[IBIS Ver]   4.0
[Comment Char] |_char
[File name]   pse84_ewlb235.ibs
[File Rev] 1.2
[Date] 10/27/2023
[Source] Infineon Technologies IBIS team
[Notes]
|Rev. 1.0 - Initial model 12/8/2021
|Rev. 1.1 - Update with RLC 8/19/2023
|Rev. 1.2 - Included pins for MIPI-DPHY DSI and USB 10/23/2023
|The temperature range is -40 to 125C.
|This model was syntax checked with Hyperlynx 4.2 visual IBIS
|editor and ibischk7_64 IBIS checker.
|There were 0 syntax errors.
[Disclaimer]   The model given below represents a 235-pin package.
[Copyright]   (C) COPYRIGHT 2023, Infineon Technologies AG.
[Component] PSOCE84
[Manufacturer] Infineon Technologies AG
| Package model eWLB235 was extracted from simulation tool.
[Package]
|   typ   min   max
R_pkg   0.27855   0.02289   0.76353
L_pkg   0.886n   0.101n   2.38n
C_pkg   0.191p   0.0717p   0.401p
[Pin]   Signal_name   model_name   R_pin   L_pin   C_pin
A10   P16_1_PAD   3p3_gpio_wbso_v 0.40002 1.87E-09   1.65E-13
A8   P17_5_PAD   3p3_gpio_wbso_v 0.60238 2.38E-09   2.00E-13
B8   P17_3_PAD   3p3_gpio_wbso_v 0.42798 1.66E-09   1.54E-13
C10   P16_3_PAD   3p3_gpio_wbso_v 0.31957 1.40E-09   1.50E-13
D7   P17_7_PAD   3p3_gpio_wbso_v 0.43638 8.69E-10   2.95E-13
E9   P16_7_PAD   3p3_gpio_wbso_v 0.45335 8.89E-10   2.99E-13
G7   P17_1_PAD   3p3_gpio_wbso_v 0.66331 1.27E-09   3.60E-13
G8   P16_5_PAD   3p3_gpio_wbso_v 0.65241 1.26E-09   3.71E-13
B10   P16_2_PAD   3p3_gpio_wbso_v 0.34579 1.53E-09   1.69E-13
B11   P16_0_PAD   3p3_gpio_wbso_v 0.28083 1.31E-09   1.32E-13
C7   P17_6_PAD   3p3_gpio_wbso_v 0.43877 1.72E-09   1.62E-13
C8   P17_4_PAD   3p3_gpio_wbso_v 0.36424 1.41E-09   1.67E-13
E7   P17_2_PAD   3p3_gpio_wbso_v 0.46653 9.28E-10   3.04E-13
E8   P17_0_PAD   3p3_gpio_wbso_v 0.39239 7.88E-10   2.83E-13
F8   P16_6_PAD   3p3_gpio_wbso_v 0.55142 1.07E-09   3.42E-13
F9   P16_4_PAD   3p3_gpio_wbso_v 0.47491 9.43E-10   3.06E-13
R10   XRES_PAD   1p8_xres_3swbso 0.029075   2.89E-10   7.84E-14
J10   P11_5_PAD   1p8_ovt_wbso_h  0.59768 1.17E-09   3.42E-13
K11   P11_3_PAD   1p8_ovt_wbso_h  0.43593 8.51E-10   3.12E-13
K12   P11_4_PAD   1p8_ovt_wbso_h  0.34228 6.90E-10   2.69E-13
K13   P11_6_PAD   1p8_ovt_wbso_h  0.24957 5.13E-10   2.42E-13
K15   P11_7_PAD   1p8_ovt_wbso_h  0.028195   1.17E-10   1.82E-13
K16   P11_1_PAD   1p8_ovt_wbso_h  0.07529 4.02E-10   7.83E-14
L11   P11_2_PAD   1p8_ovt_wbso_h  0.43058 8.35E-10   3.10E-13
L16   P11_0_PAD   1p8_ovt_wbso_h  0.02734 1.88E-10   7.18E-14
H7   P3_0_PAD   1p8_ioi3c_3swbso_h   0.39265 8.57E-10   3.36E-13
H8   P3_1_PAD   1p8_ioi3c_3swbso_h   0.46598 1.05E-09   3.57E-13
A14   P20_4_PAD   1p8_ioi2c_wbso_h   0.23793 1.20E-09   1.02E-13
B12   P20_6_PAD   1p8_ioi2c_wbso_h   0.18255 9.43E-10   9.44E-14
B14   P20_2_PAD   1p8_ioi2c_wbso_h   0.14411 7.56E-10   8.93E-14
B15   P20_0_PAD   1p8_ioi2c_wbso_h   0.1456  7.01E-10   9.21E-14
E12   P9_2_PAD   1p8_ioi2c_wbso_h   0.25292 5.97E-10   2.66E-13
F10   P9_0_PAD   1p8_ioi2c_wbso_h   0.66966 1.28E-09   3.71E-13
K9   P8_7_PAD   1p8_ioi2c_wbso_h   0.47076 9.33E-10   3.06E-13
M8   P8_6_PAD   1p8_ioi2c_wbso_h   0.21737 4.56E-10   2.33E-13
R8   P8_2_PAD   1p8_ioi2c_wbso_h   0.039885 3.42E-10   7.77E-14
T6   P8_4_PAD   1p8_ioi2c_wbso_h   0.36053 1.26E-09   1.31E-13
T7   P8_5_PAD   1p8_ioi2c_wbso_h   0.17838 7.65E-10   9.60E-14
U6   P8_3_PAD   1p8_ioi2c_wbso_h   0.40499 1.49E-09   1.31E-13
A2   P6_4_PAD   1p8_ioi2c_wbso_h   0.31511 1.29E-09   1.19E-13
B2   P6_6_PAD   1p8_ioi2c_wbso_h   0.2468  1.02E-09   1.15E-13
K8   P21_4_PAD   1p8_ioi2c_wbso_h   0.6339  1.22E-09   3.78E-13
L12   P10_1_PAD   1p8_ioi2c_wbso_h   0.2568  6.95E-10   3.15E-13
M15   P10_2_PAD   1p8_ioi2c_wbso_h   0.022894 1.01E-10   1.82E-13
M4   P21_6_PAD   1p8_ioi2c_wbso_h   0.089229 2.15E-10   1.97E-13
P16   P10_3_PAD   1p8_ioi2c_wbso_h   0.31745 1.26E-09   1.37E-13
P4   P12_0_PAD   1p8_ioi2c_wbso_h   0.083721 2.60E-10   2.03E-13
R2   P21_2_PAD   1p8_ioi2c_wbso_h   0.29537 1.18E-09   1.23E-13
T16   P10_0_PAD   1p8_ioi2c_wbso_h   0.26089 1.05E-09   1.83E-13
T2   P21_0_PAD   1p8_ioi2c_wbso_h   0.37991 1.33E-09   1.56E-13
T3   P12_2_PAD   1p8_ioi2c_wbso_h   0.22827 9.38E-10   1.27E-13
U2   P12_4_PAD   1p8_ioi2c_wbso_h   0.34327 1.27E-09   1.28E-13
A12   P20_5_PAD   1p8_ioi2c_wbso_h   0.27304 1.32E-09   1.10E-13
A16   P20_1_PAD   1p8_ioi2c_wbso_h   0.31259 1.50E-09   1.18E-13
C12   P20_7_PAD   1p8_ioi2c_wbso_h   0.15854 7.92E-10   9.47E-14
C14   P20_3_PAD   1p8_ioi2c_wbso_h   0.064528 3.41E-10   8.12E-14
F11   P9_1_PAD   1p8_ioi2c_wbso_h   0.48015 9.35E-10   3.18E-13
G9   P9_3_PAD   1p8_ioi2c_wbso_h   0.71533 1.38E-09   3.75E-13
B1   P6_7_PAD   1p8_ioi2c_wbso_h   0.35877 1.34E-09   1.24E-13
B3   P6_5_PAD   1p8_ioi2c_wbso_h   0.22409 8.52E-10   1.02E-13
L7   P21_7_PAD   1p8_ioi2c_wbso_h   0.39102 7.76E-10   2.88E-13
L8   P21_3_PAD   1p8_ioi2c_wbso_h   0.5432  1.04E-09   3.65E-13
M5   P21_5_PAD   1p8_ioi2c_wbso_h   0.19144 3.96E-10   2.31E-13
R3   P12_5_PAD   1p8_ioi2c_wbso_h   0.066979 4.06E-10   8.45E-14
R4   P12_1_PAD   1p8_ioi2c_wbso_h   0.15282 5.87E-10   1.11E-13
T1   P21_1_PAD   1p8_ioi2c_wbso_h   0.4827  1.76E-09   1.69E-13
U3   P12_3_PAD   1p8_ioi2c_wbso_h   0.30929 1.38E-09   1.36E-13
A3   P6_3_PAD   1p8_ioi2c_wbso_h   0.17141 1.04E-09   1.16E-13
A4   P6_2_PAD   1p8_ioi2c_wbso_h   0.17085 1.05E-09   1.16E-13
B4   P6_1_PAD   1p8_ioi2c_wbso_h   0.1086  6.90E-10   8.90E-14
C6   P6_0_PAD   1p8_ioi2c_wbso_h   0.16176 7.51E-10   1.29E-13
K10   P8_0_PAD   1p8_ioi2c_wbso_h   0.60411 1.17E-09   3.43E-13
T8   P8_1_PAD   1p8_ioi2c_wbso_h   0.093729 6.77E-10   9.47E-14
B17   P15_6_PAD   1p8_ioi2c_wbso_h   0.20398 1.14E-09   1.22E-13
C16   P15_7_PAD   1p8_ioi2c_wbso_h   0.067252 4.46E-10   9.19E-14
D17   P15_5_PAD   1p8_ioi2c_wbso_h   0.070339 5.96E-10   8.57E-14
D5   P7_0_PAD   1p8_ioi2c_wbso_h   0.11478 3.74E-10   2.53E-13
D6   P7_1_PAD   1p8_ioi2c_wbso_h   0.16742 5.37E-10   2.92E-13
E13   P15_2_PAD   1p8_ioi2c_wbso_h   0.25733 5.38E-10   2.45E-13
E14   P15_4_PAD   1p8_ioi2c_wbso_h   0.081059 2.78E-10   2.26E-13
E15   P15_3_PAD   1p8_ioi2c_wbso_h   0.025532 1.19E-10   1.83E-13
E4   P7_3_PAD   1p8_ioi2c_wbso_h   0.055855 2.08E-10   2.06E-13
E5   P7_2_PAD   1p8_ioi2c_wbso_h   0.11743 3.88E-10   2.55E-13
E6   P7_4_PAD   1p8_ioi2c_wbso_h   0.24242 5.86E-10   2.61E-13
F12   P14_7_PAD   1p8_ioi2c_wbso_h   0.34149 6.90E-10   2.68E-13
F5   P7_7_PAD   1p8_ioi2c_wbso_h   0.17069 4.12E-10   2.35E-13
F6   P7_6_PAD   1p8_ioi2c_wbso_h   0.24699 5.83E-10   2.64E-13
F7   P7_5_PAD   1p8_ioi2c_wbso_h   0.32363 7.53E-10   2.94E-13
G10   P15_1_PAD   1p8_ioi2c_wbso_h   0.61435 1.19E-09   3.59E-13
G11   P15_0_PAD   1p8_ioi2c_wbso_h   0.51504 1.01E-09   3.30E-13
G13   P14_1_PAD   1p8_ioi2c_wbso_h   0.24567 5.08E-10   2.41E-13
G14   P14_2_PAD   1p8_ioi2c_wbso_h   0.15156 3.32E-10   2.14E-13
G15   P14_4_PAD   1p8_ioi2c_wbso_h   0.026776 1.16E-10   1.82E-13
G16   P14_3_PAD   1p8_ioi2c_wbso_h   0.024953 2.04E-10   7.17E-14
H11   P13_4_PAD   1p8_ioi2c_wbso_h   0.54528 1.07E-09   3.27E-13
H15   P13_7_PAD   1p8_ioi2c_wbso_h   0.027337 1.27E-10   1.83E-13
H16   P13_6_PAD   1p8_ioi2c_wbso_h   0.025252 2.17E-10   7.17E-14
H17   P13_3_PAD   1p8_ioi2c_wbso_h   0.087473 6.10E-10   8.99E-14
H9   P14_6_PAD   1p8_ioi2c_wbso_h   0.68922 1.33E-09   3.79E-13
J15   P13_1_PAD   1p8_ioi2c_wbso_h   0.027158 1.27E-10   1.82E-13
K17   P13_2_PAD   1p8_ioi2c_wbso_h   0.094103 6.86E-10   8.97E-14
L13   P10_5_PAD   1p8_ioi2c_wbso_h   0.1588  4.46E-10   2.58E-13
M17   P10_7_PAD   1p8_ioi2c_wbso_h   0.14888 6.24E-10   9.27E-14
P17   P10_6_PAD   1p8_ioi2c_wbso_h   0.32481 1.30E-09   1.33E-13
T17   P10_4_PAD   1p8_ioi2c_wbso_h   0.51391 1.97E-09   1.78E-13
K7   P0_0_PAD   1p8_hsio_wbso_h 0.48364 9.47E-10   3.26E-13
L6   P0_1_PAD   1p8_hsio_wbso_h 0.28925 5.78E-10   2.85E-13
J7   P2_0_PAD   1p8_hsio_wbso_h 0.32813 7.58E-10   2.96E-13
J8   P5_0_PAD   1p8_hsio_wbso_h 0.24691 7.60E-10   3.60E-13
R9   P18_0_PAD   1p8_gpib_3swbso_h   0.040604 3.56E-10   8.06E-14
T10   P19_1_PAD   1p8_gpib_3swbso_h   0.17473 7.57E-10   1.02E-13
T9   P18_1_PAD   1p8_gpib_3swbso_h   0.17546 7.69E-10   1.03E-13
U8   P19_0_PAD   1p8_gpib_3swbso_h   0.36835 1.50E-09   1.33E-13
G12   P14_0_PAD   1p8_gpib_3swbso_h   0.33937 6.91E-10   2.68E-13
H10   P13_0_PAD   1p8_gpib_3swbso_h   0.47458 1.07E-09   3.58E-13
H12   P13_5_PAD   1p8_gpib_3swbso_h   0.44709 8.82E-10   2.99E-13
J9   P14_5_PAD   1p8_gpib_3swbso_h   0.76353 1.46E-09   4.01E-13
B16   VDDIO_2_PAD   POWER
C3   VDDIO_0_PAD   POWER
C5   VDD33_USB_PAD   POWER
D8   VCCD_3_PAD   POWER
E10   VDDIO_1P8_3P3_PAD   POWER
E11   VDDP_PAD   POWER
E2   VDDIO_SMIF0_1_PAD   POWER
F13   VDDA_SAR_PAD   POWER
F14   VDDA_PAD   POWER
F16   VDDIO_A_Q_PAD   POWER
F17   VREF_PAD   POWER
F4   VCCSRAMI_1_PAD  POWER
G5   VDDIO_SMIF0_0_PAD   POWER
H13   VDDA_CTB_PAD   POWER
H6   VDDIO_SMIF0_2_PAD   POWER
J11   VCCD_1_PAD   POWER
J12   VCCSRAMI_0_PAD  POWER
J14   VDDIO_A_PAD   POWER
J5   VCCD_0_PAD   POWER
J6   VDDD_DLL_PAD   POWER
K4   VDDIO_SMIF1_2_PAD   POWER
L10   VDDPUMP_RRAM_PAD   POWER
L14   VDDIO_3_PAD   POWER
L5   VDDIO_SMIF1_1_PAD   POWER
L9   VDDIO_1_PAD   POWER
M10   VDDD_PAD   POWER
M11   VCCIRETLDO_PAD  POWER
M12   VDDQ_SR1P8_PAD  POWER
M13   VDDQ_0_PAD   POWER
M14   VDDLX_SR_PAD   POWER
M6   VP_DSI_PAD   POWER
M7   VPL_P_DSI_PAD   POWER
M9   VDDIO_CO_PAD   POWER
N10   VCCD_ANA_PAD   POWER
N11   VCCSRAM_PAD   POWER
N12   VCCRET_PAD   POWER
N13   VDDBAT_SR_PAD   POWER
N15   VCCI_SR1P8_0_PAD   POWER
N2   VDDIO_SMIF1_0_PAD   POWER
N4   VCCD_4_PAD   POWER
N7   VPH_P_DSI_PAD   POWER
P5   VDDIO_4_PAD   POWER
R11   VDDDLDO_PAD   POWER
R13   VDDBAT_0_PAD   POWER
R14   VCCI_SR_0_PAD   POWER
R15   VDDD_SR1P8_PAD  POWER
R16   VDDLX_SR1P8_PAD POWER
T12   VDDQ_SR_PAD   POWER
T13   VDDD_SR_PAD   POWER
T15   VDDD_SR1P8_PAD  POWER
U11   VCCD_2_PAD   POWER
U12   VDDQ_SR_PAD   POWER
U13   VDDD_SR_PAD   POWER
|A6   USB_DM_PAD   PAD 0.17731 1.28E-09   1.12E-13
|B6   USB_DP_PAD   PAD 0.13288 9.73E-10   1.01E-13
D1   SMIF0_SPIHB_CLK_P_PAD   Mpad_0  0.50222 1.72E-09   1.73E-13
E1   SMIF0_SPIHB_CLK_N_PAD   Mpad_0  0.42165 1.47E-09   1.44E-13
H5   SMIF0_SPIHB_RWDS_PAD   Mpad   0.10126 3.22E-10   2.42E-13
K6   SMIF1_SPIHB_RWDS_PAD   Mpad   0.17656 4.90E-10   2.67E-13
M1   SMIF1_SPIHB_CLK_N_PAD   Mpad_0  0.39766 1.56E-09   1.53E-13
N1   SMIF1_SPIHB_CLK_P_PAD   Mpad_1  0.37923 1.51E-09   1.64E-13
|N6   DSI_REXT_PAD   PAD   0.057605   2.02E-10   2.07E-13
|R5   DSI_DATA0_P_PAD PAD   0.099446   4.95E-10   1.03E-13
|R6   DSI_DATA0_N_PAD PAD   0.037035   3.03E-10   7.63E-14
|T4   DSI_DATA1_P_PAD PAD   0.18387 1.02E-09   1.18E-13
|T5   DSI_DATA1_N_PAD PAD   0.12513 7.85E-10   9.78E-14
|U4   DSI_CLK_N_PAD   PAD   0.31139 1.65E-09   1.56E-13
|U5   DSI_CLK_P_PAD   PAD   0.18664 1.13E-09   1.14E-13
A1   VSSD   GND
A17   VSSD   GND
C11   VSSD   GND
C15   VSSD   GND
C2   VSSD   GND
C4   VSS_USB_PAD   GND
D16   VSSA   GND
D9   VSSD   GND
F15   VSSA   GND
G4   VSSD   GND
G6   VSSD   GND
H14   VSSA   GND
J13   VSSA   GND
J4   VSSD   GND
K14   VSSD   GND
K5   VSSD   GND
L15   VSSD   GND
L4   VSSD   GND
M16   VSSD   GND
N14   VSS_SR_PAD   GND
N16   VSS_SR1P8_PAD   GND
N5   VSSD   GND
N8   VSSD   GND
N9   VSSD   GND
R12   VSSQ_PAD   GND
R7   VSSD   GND
T11   VSSQ_PAD   GND
T14   VSSD   GND
U1   VSSD   GND
U10   VSSD   GND
U14   VSSQ_PAD   GND
U15   VSSQ_PAD   GND
U16   VSSQ_PAD   GND
U17   VSSD   GND
C1   SMIF0_SPIHB_DATA3_PAD   Mpad   0.64588  1.93E-09   1.93E-13
D2   SMIF0_SPIHB_DATA2_PAD   Mpad   0.56889  1.71E-09   1.62E-13
F1   SMIF0_SPIHB_DATA6_PAD   Mpad   0.46139  1.70E-09   1.59E-13
F2   SMIF0_SPIHB_DATA0_PAD   Mpad   0.066223 4.38E-10   8.92E-14
G1   SMIF0_SPIHB_DATA5_PAD   Mpad   0.29133  1.20E-09   1.19E-13
G2   SMIF0_SPIHB_DATA1_PAD   Mpad   0.089554 3.98E-10   8.20E-14
H2   SMIF0_SPIHB_DATA4_PAD   Mpad   0.10035  4.45E-10   8.32E-14
H4   SMIF0_SPIHB_DATA7_PAD   Mpad   0.044798 1.60E-10   1.96E-13
J1   SMIF1_SPIHB_DATA5_PAD   Mpad   0.21445  1.09E-09   9.82E-14
J2   SMIF1_SPIHB_DATA7_PAD   Mpad   0.086738 5.38E-10   8.81E-14
K1   SMIF1_SPIHB_DATA4_PAD   Mpad   0.2036   8.48E-10   9.45E-14
K2   SMIF1_SPIHB_DATA6_PAD   Mpad   0.062656 3.86E-10   8.27E-14
L2   SMIF1_SPIHB_DATA2_PAD   Mpad   0.06289  3.78E-10   8.25E-14
M2   SMIF1_SPIHB_DATA0_PAD   Mpad   0.059779 4.41E-10   8.82E-14
P2   SMIF1_SPIHB_DATA1_PAD   Mpad   0.42174  1.40E-09   1.44E-13
R1   SMIF1_SPIHB_DATA3_PAD   Mpad   0.55987  2.16E-09   1.77E-13
[Diff_pin]   inv_pin   vdiff   tdelay_typ   tdelay_min   tdelay_max
D1   E1   0.2   -40.2244p   NA   NA
N1   M1   0.2   -40.2244p   NA   NA
|***   MODEL SELECTOR   ***
[Model Selector] 1p8_hsio_wbso_h
| Model Description
hsio_drive000_slew0  obuf mode with drive_sel=000 and slew_sel=0
hsio_drive000_slew1  obuf mode with drive_sel=000 and slew_sel=1
hsio_drive001_slew0  obuf mode with drive_sel=001 and slew_sel=0
hsio_drive001_slew1  obuf mode with drive_sel=001 and slew_sel=1
hsio_drive010_slew0  obuf mode with drive_sel=010 and slew_sel=0
hsio_drive010_slew1  obuf mode with drive_sel=010 and slew_sel=1
hsio_drive011_slew0  obuf mode with drive_sel=011 and slew_sel=0
hsio_drive011_slew1  obuf mode with drive_sel=011 and slew_sel=1
hsio_drive100_slew0  obuf mode with drive_sel=100 and slew_sel=0
hsio_drive100_slew1  obuf mode with drive_sel=100 and slew_sel=1
hsio_drive101_slew0  obuf mode with drive_sel=101 and slew_sel=0
hsio_drive101_slew1  obuf mode with drive_sel=101 and slew_sel=1
hsio_drive110_slew0  obuf mode with drive_sel=110 and slew_sel=0
hsio_drive110_slew1  obuf mode with drive_sel=110 and slew_sel=1
hsio_drive111_slew0  obuf mode with drive_sel=111 and slew_sel=0
hsio_drive111_slew1  obuf mode with drive_sel=111 and slew_sel=1
[Model Selector] 1p8_ioi2c_wbso_h
| Model Description
ioi2c_drive000_slew0   obuf mode with drive_sel=000 and slew_sel=0
ioi2c_drive000_slew1   obuf mode with drive_sel=000 and slew_sel=1
ioi2c_drive100_slew0   obuf mode with drive_sel=100 and slew_sel=0
ioi2c_drive100_slew1   obuf mode with drive_sel=100 and slew_sel=1
ioi2c_drive010_slew0   obuf mode with drive_sel=010 and slew_sel=0
ioi2c_drive010_slew1   obuf mode with drive_sel=010 and slew_sel=1
ioi2c_drive110_slew0   obuf mode with drive_sel=110 and slew_sel=0
ioi2c_drive110_slew1   obuf mode with drive_sel=110 and slew_sel=1
ioi2c_drive001_slew0   obuf mode with drive_sel=001 and slew_sel=0
ioi2c_drive001_slew1   obuf mode with drive_sel=001 and slew_sel=1
ioi2c_drive101_slew0   obuf mode with drive_sel=101 and slew_sel=0
ioi2c_drive101_slew1   obuf mode with drive_sel=101 and slew_sel=1
ioi2c_drive011_slew0   obuf mode with drive_sel=011 and slew_sel=0
ioi2c_drive011_slew1   obuf mode with drive_sel=011 and slew_sel=1
ioi2c_drive111_slew0   obuf mode with drive_sel=111 and slew_sel=0
ioi2c_drive111_slew1   obuf mode with drive_sel=111 and slew_sel=1
ioi2c_drive000_slow1   obuf mode with drive_sel=000 and slow=1
ioi2c_drive100_slow1   obuf mode with drive_sel=100 and slow=1
ioi2c_drive010_slow1   obuf mode with drive_sel=010 and slow=1
ioi2c_drive110_slow1   obuf mode with drive_sel=110 and slow=1
ioi2c_drive001_slow1   obuf mode with drive_sel=001 and slow=1
ioi2c_drive101_slow1   obuf mode with drive_sel=101 and slow=1
ioi2c_drive011_slow1   obuf mode with drive_sel=011 and slow=1
ioi2c_drive111_slow1   obuf mode with drive_sel=111 and slow=1
[Model Selector] 1p8_ioi3c_3swbso_h
| Model Description
ioi3c_drive000_slew0   obuf mode with drive_sel=000 and slew_sel=0
ioi3c_drive000_slew1   obuf mode with drive_sel=000 and slew_sel=1
ioi3c_drive100_slew0   obuf mode with drive_sel=100 and slew_sel=0
ioi3c_drive100_slew1   obuf mode with drive_sel=100 and slew_sel=1
ioi3c_drive010_slew0   obuf mode with drive_sel=010 and slew_sel=0
ioi3c_drive010_slew1   obuf mode with drive_sel=010 and slew_sel=1
ioi3c_drive110_slew0   obuf mode with drive_sel=110 and slew_sel=0
ioi3c_drive110_slew1   obuf mode with drive_sel=110 and slew_sel=1
ioi3c_drive001_slew0   obuf mode with drive_sel=001 and slew_sel=0
ioi3c_drive001_slew1   obuf mode with drive_sel=001 and slew_sel=1
ioi3c_drive101_slew0   obuf mode with drive_sel=101 and slew_sel=0
ioi3c_drive101_slew1   obuf mode with drive_sel=101 and slew_sel=1
ioi3c_drive011_slew0   obuf mode with drive_sel=011 and slew_sel=0
ioi3c_drive011_slew1   obuf mode with drive_sel=011 and slew_sel=1
ioi3c_drive111_slew0   obuf mode with drive_sel=111 and slew_sel=0
ioi3c_drive111_slew1   obuf mode with drive_sel=111 and slew_sel=1
ioi3c_drive000_slow1   obuf mode with drive_sel=000 and slow=1
ioi3c_drive100_slow1   obuf mode with drive_sel=100 and slow=1
ioi3c_drive010_slow1   obuf mode with drive_sel=010 and slow=1
ioi3c_drive110_slow1   obuf mode with drive_sel=110 and slow=1
ioi3c_drive001_slow1   obuf mode with drive_sel=001 and slow=1
ioi3c_drive101_slow1   obuf mode with drive_sel=101 and slow=1
ioi3c_drive011_slow1   obuf mode with drive_sel=011 and slow=1
ioi3c_drive111_slow1   obuf mode with drive_sel=111 and slow=1
[Model Selector] 1p8_ovt_wbso_h
| Model Description
ovt_000_slew0   obuf mode with drive_sel=000 and slew_sel=0
ovt_000_slew1   obuf mode with drive_sel=000 and slew_sel=1
ovt_100_slew0   obuf mode with drive_sel=100 and slew_sel=0
ovt_100_slew1   obuf mode with drive_sel=100 and slew_sel=1
ovt_010_slew0   obuf mode with drive_sel=010 and slew_sel=0
ovt_010_slew1   obuf mode with drive_sel=010 and slew_sel=1
ovt_110_slew0   obuf mode with drive_sel=110 and slew_sel=0
ovt_110_slew1   obuf mode with drive_sel=110 and slew_sel=1
ovt_001_slew0   obuf mode with drive_sel=001 and slew_sel=0
ovt_001_slew1   obuf mode with drive_sel=001 and slew_sel=1
ovt_101_slew0   obuf mode with drive_sel=101 and slew_sel=0
ovt_101_slew1   obuf mode with drive_sel=101 and slew_sel=1
ovt_011_slew0   obuf mode with drive_sel=011 and slew_sel=0
ovt_011_slew1   obuf mode with drive_sel=011 and slew_sel=1
ovt_111_slew0   obuf mode with drive_sel=111 and slew_sel=0
ovt_111_slew1   obuf mode with drive_sel=111 and slew_sel=1
ovt_000_slow1   obuf mode with drive_sel=000 and slow=1
ovt_100_slow1   obuf mode with drive_sel=100 and slow=1
ovt_010_slow1   obuf mode with drive_sel=010 and slow=1
ovt_110_slow1   obuf mode with drive_sel=110 and slow=1
ovt_001_slow1   obuf mode with drive_sel=001 and slow=1
ovt_101_slow1   obuf mode with drive_sel=101 and slow=1
ovt_011_slow1   obuf mode with drive_sel=011 and slow=1
ovt_111_slow1   obuf mode with drive_sel=111 and slow=1
[Model Selector] 3p3_gpio_wbso_v
| Model Description
gpio_000_slew0_slow0   obuf mode with drive_sel=000 and slew_sel=0
gpio_000_slew1_slow0   obuf mode with drive_sel=000 and slew_sel=1
gpio_100_slew0_slow0   obuf mode with drive_sel=100 and slew_sel=0
gpio_100_slew1_slow0   obuf mode with drive_sel=100 and slew_sel=1
gpio_010_slew0_slow0   obuf mode with drive_sel=010 and slew_sel=0
gpio_010_slew1_slow0   obuf mode with drive_sel=010 and slew_sel=1
gpio_110_slew0_slow0   obuf mode with drive_sel=110 and slew_sel=0
gpio_110_slew1_slow0   obuf mode with drive_sel=110 and slew_sel=1
gpio_001_slew0_slow0   obuf mode with drive_sel=001 and slew_sel=0
gpio_001_slew1_slow0   obuf mode with drive_sel=001 and slew_sel=1
gpio_101_slew0_slow0   obuf mode with drive_sel=101 and slew_sel=0
gpio_101_slew1_slow0   obuf mode with drive_sel=101 and slew_sel=1
gpio_011_slew0_slow0   obuf mode with drive_sel=011 and slew_sel=0
gpio_011_slew1_slow0   obuf mode with drive_sel=011 and slew_sel=1
gpio_111_slew0_slow0   obuf mode with drive_sel=111 and slew_sel=0
gpio_111_slew1_slow0   obuf mode with drive_sel=111 and slew_sel=1
gpio_000_slew0_slow1   obuf mode with drive_sel=000 for slow=1 and slew=0
gpio_000_slew1_slow1   obuf mode with drive_sel=000 for slow=1 and slew=1
gpio_100_slew0_slow1   obuf mode with drive_sel=100 for slow=1 and slew=0
gpio_100_slew1_slow1   obuf mode with drive_sel=100 for slow=1 and slew=1
gpio_010_slew0_slow1   obuf mode with drive_sel=010 for slow=1 and slew=0
gpio_010_slew1_slow1   obuf mode with drive_sel=010 for slow=1 and slew=1
gpio_110_slew0_slow1   obuf mode with drive_sel=110 for slow=1 and slew=0
gpio_110_slew1_slow1   obuf mode with drive_sel=110 for slow=1 and slew=1
gpio_001_slew0_slow1   obuf mode with drive_sel=001 for slow=1 and slew=0
gpio_001_slew1_slow1   obuf mode with drive_sel=001 for slow=1 and slew=1
gpio_101_slew0_slow1   obuf mode with drive_sel=101 for slow=1 and slew=0
gpio_101_slew1_slow1   obuf mode with drive_sel=101 for slow=1 and slew=1
gpio_011_slew0_slow1   obuf mode with drive_sel=011 for slow=1 and slew=0
gpio_011_slew1_slow1   obuf mode with drive_sel=011 for slow=1 and slew=1
gpio_111_slew0_slow1   obuf mode with drive_sel=111 for slow=1 and slew=0
gpio_111_slew1_slow1   obuf mode with drive_sel=111 for slow=1 and slew=1
| pad
[Model Selector] Mpad
| Model Description
hsio_drive000_slew0  obuf mode with drive_sel=000 and slew_sel=0
hsio_drive000_slew1  obuf mode with drive_sel=000 and slew_sel=1
hsio_drive001_slew0  obuf mode with drive_sel=001 and slew_sel=0
hsio_drive001_slew1  obuf mode with drive_sel=001 and slew_sel=1
hsio_drive010_slew0  obuf mode with drive_sel=010 and slew_sel=0
hsio_drive010_slew1  obuf mode with drive_sel=010 and slew_sel=1
hsio_drive011_slew0  obuf mode with drive_sel=011 and slew_sel=0
hsio_drive011_slew1  obuf mode with drive_sel=011 and slew_sel=1
hsio_drive100_slew0  obuf mode with drive_sel=100 and slew_sel=0
hsio_drive100_slew1  obuf mode with drive_sel=100 and slew_sel=1
hsio_drive101_slew0  obuf mode with drive_sel=101 and slew_sel=0
hsio_drive101_slew1  obuf mode with drive_sel=101 and slew_sel=1
hsio_drive110_slew0  obuf mode with drive_sel=110 and slew_sel=0
hsio_drive110_slew1  obuf mode with drive_sel=110 and slew_sel=1
hsio_drive111_slew0  obuf mode with drive_sel=111 and slew_sel=0
hsio_drive111_slew1  obuf mode with drive_sel=111 and slew_sel=1
[Model Selector] Mpad_0
| Model Description
p0_drive000_slew0  obuf mode with drive_sel=000 and slew_sel=0
p0_drive000_slew1  obuf mode with drive_sel=000 and slew_sel=1
p0_drive001_slew0  obuf mode with drive_sel=001 and slew_sel=0
p0_drive001_slew1  obuf mode with drive_sel=001 and slew_sel=1
p0_drive010_slew0  obuf mode with drive_sel=010 and slew_sel=0
p0_drive010_slew1  obuf mode with drive_sel=010 and slew_sel=1
p0_drive011_slew0  obuf mode with drive_sel=011 and slew_sel=0
p0_drive011_slew1  obuf mode with drive_sel=011 and slew_sel=1
p0_drive100_slew0  obuf mode with drive_sel=100 and slew_sel=0
p0_drive100_slew1  obuf mode with drive_sel=100 and slew_sel=1
p0_drive101_slew0  obuf mode with drive_sel=101 and slew_sel=0
p0_drive101_slew1  obuf mode with drive_sel=101 and slew_sel=1
p0_drive110_slew0  obuf mode with drive_sel=110 and slew_sel=0
p0_drive110_slew1  obuf mode with drive_sel=110 and slew_sel=1
p0_drive111_slew0  obuf mode with drive_sel=111 and slew_sel=0
p0_drive111_slew1  obuf mode with drive_sel=111 and slew_sel=1
[Model Selector] Mpad_1
| Model Description
p1_drive000_slew0  obuf mode with drive_sel=000 and slew_sel=0
p1_drive000_slew1  obuf mode with drive_sel=000 and slew_sel=1
p1_drive001_slew0  obuf mode with drive_sel=001 and slew_sel=0
p1_drive001_slew1  obuf mode with drive_sel=001 and slew_sel=1
p1_drive010_slew0  obuf mode with drive_sel=010 and slew_sel=0
p1_drive010_slew1  obuf mode with drive_sel=010 and slew_sel=1
p1_drive011_slew0  obuf mode with drive_sel=011 and slew_sel=0
p1_drive011_slew1  obuf mode with drive_sel=011 and slew_sel=1
p1_drive100_slew0  obuf mode with drive_sel=100 and slew_sel=0
p1_drive100_slew1  obuf mode with drive_sel=100 and slew_sel=1
p1_drive101_slew0  obuf mode with drive_sel=101 and slew_sel=0
p1_drive101_slew1  obuf mode with drive_sel=101 and slew_sel=1
p1_drive110_slew0  obuf mode with drive_sel=110 and slew_sel=0
p1_drive110_slew1  obuf mode with drive_sel=110 and slew_sel=1
p1_drive111_slew0  obuf mode with drive_sel=111 and slew_sel=0
p1_drive111_slew1  obuf mode with drive_sel=111 and slew_sel=1
| Models and submodels in the file (154): 1p8_gpib_3swbso_h (Input), ioi2c_drive000_slew0 (I/O), ioi2c_drive000_slew1 (I/O), ioi2c_drive100_slew0 (I/O), ioi2c_drive100_slew1 (I/O), ioi2c_drive010_slew0 (I/O), ioi2c_drive010_slew1 (I/O), ioi2c_drive110_slew0 (I/O), ioi2c_drive110_slew1 (I/O), ioi2c_drive001_slew0 (I/O), ioi2c_drive001_slew1 (I/O), ioi2c_drive101_slew0 (I/O), ioi2c_drive101_slew1 (I/O), ioi2c_drive011_slew0 (I/O), ioi2c_drive011_slew1 (I/O), ioi2c_drive111_slew0 (I/O), ioi2c_drive111_slew1 (I/O), ioi2c_drive000_slow1 (I/O), ioi2c_drive100_slow1 (I/O), ioi2c_drive010_slow1 (I/O), ioi2c_drive110_slow1 (I/O), ioi2c_drive001_slow1 (I/O), ioi2c_drive101_slow1 (I/O), ioi2c_drive011_slow1 (I/O), ioi2c_drive111_slow1 (I/O), ioi3c_drive000_slew0 (I/O), ioi3c_drive000_slew1 (I/O), ioi3c_drive100_slew0 (I/O), ioi3c_drive100_slew1 (I/O), ioi3c_drive010_slew0 (I/O), ioi3c_drive010_slew1 (I/O), ioi3c_drive110_slew0 (I/O), ioi3c_drive110_slew1 (I/O), ioi3c_drive001_slew0 (I/O), ioi3c_drive001_slew1 (I/O), ioi3c_drive101_slew0 (I/O), ioi3c_drive101_slew1 (I/O), ioi3c_drive011_slew0 (I/O), ioi3c_drive011_slew1 (I/O), ioi3c_drive111_slew0 (I/O), ioi3c_drive111_slew1 (I/O), ioi3c_drive000_slow1 (I/O), ioi3c_drive100_slow1 (I/O), ioi3c_drive010_slow1 (I/O), ioi3c_drive110_slow1 (I/O), ioi3c_drive001_slow1 (I/O), ioi3c_drive101_slow1 (I/O), ioi3c_drive011_slow1 (I/O), ioi3c_drive111_slow1 (I/O), ovt_000_slew0 (I/O), ovt_000_slew1 (I/O), ovt_100_slew0 (I/O), ovt_100_slew1 (I/O), ovt_010_slew0 (I/O), ovt_010_slew1 (I/O), ovt_110_slew0 (I/O), ovt_110_slew1 (I/O), ovt_001_slew0 (I/O), ovt_001_slew1 (I/O), ovt_101_slew0 (I/O), ovt_101_slew1 (I/O), ovt_011_slew0 (I/O), ovt_011_slew1 (I/O), ovt_111_slew0 (I/O), ovt_111_slew1 (I/O), ovt_000_slow1 (I/O), ovt_100_slow1 (I/O), ovt_010_slow1 (I/O), ovt_110_slow1 (I/O), ovt_001_slow1 (I/O), ovt_101_slow1 (I/O), ovt_011_slow1 (I/O), ovt_111_slow1 (I/O), 1p8_xres_3swbso (Input), gpio_000_slew0_slow0 (I/O), gpio_000_slew1_slow0 (I/O), gpio_100_slew0_slow0 (I/O), gpio_100_slew1_slow0 (I/O), gpio_010_slew0_slow0 (I/O), gpio_010_slew1_slow0 (I/O)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
